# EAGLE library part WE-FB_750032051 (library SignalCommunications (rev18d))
WE-FB 3751 Flyback Transformer for LT3751 Characteristics Isolation voltage: 1 kVAC Operating temperature: –40 ºC to +125 ºC (incl. self-heating) Especially designed for LT3751 Applications Transformer for capacitor charger or high voltage outputs Details see: http://katalog.we-online.de/en/pbs/WE-FB-3751 Updated 2015-04-03 2015 (C) Wurth Elektronik
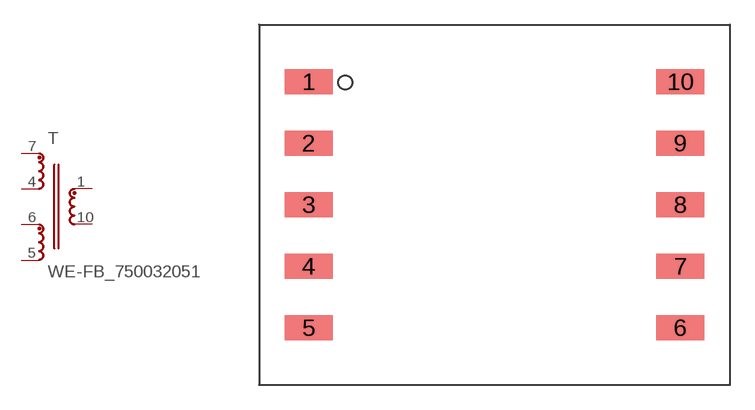
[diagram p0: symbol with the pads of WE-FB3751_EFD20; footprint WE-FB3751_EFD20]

Designator prefix T

## WE-FB_750032051  [WE-FB3751_EFD20]
1  2  pas
4  6  pas
5  4  pas
6  5  pas
7  1  pas
10  3  pas

## Footprint WE-FB3751_EFD20 (pad centres in mm)
smd 2.92 x 1.52: 1 -11.33,7.5; 2 -11.33,3.75; 3 -11.33,0; 4 -11.33,-3.75; 5 -11.33,-7.5; 6 11.33,-7.5; 7 11.33,-3.75; 8 11.33,0; 9 11.33,3.75; 10 11.33,7.5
